PROGRAM MAIN_Simu
VAR
	bReset						AT %I*: BOOL;
(***** Cylinder states *****)
	bClampAtBase				AT %Q*: BOOL;					// True if clamp cylinder is in base position
	bClampAtWork				AT %Q*: BOOL;					// True if clamp cylinder is in work position
	bBarrierAtBase				AT %Q*: BOOL;					// True if barrier cylinder is in base position
	bBarrierAtWork				AT %Q*: BOOL;					// True if barrier cylinder is in work position
	bMetalAtBase				AT %Q*: BOOL;					// True if metal cylinder is in base position
	bMetalAtWork				AT %Q*: BOOL;					// True if metal cylinder is in work position
	bPlasticAtBase				AT %Q*: BOOL;					// True if plastic cylinder is in base position
	bPlasticAtWork				AT %Q*: BOOL;					// True if plastic cylinder is in work position
(***** Temperatures *****)
	lrClampTempCurrent			AT %Q*: LREAL;					// Current temperature of clamp cylinder
	lrClampTempMax				AT %Q*: LREAL;					// Maximum temperature of clamp cylinder
	lrClampTempMin				AT %Q*: LREAL;					// Minimum temperature of clamp cylinder
	lrBarrierTemp				AT %Q*: LREAL;					// Temperature of barrier cylinder

(***** Sensors to detect boxes *****)
	bBarrierSensor				AT %Q*: BOOL;					// True if barrier sensor detects a box
	bMetalSensor				AT %Q*: BOOL;					// True if metal sensor detects a metal box
	bPlasticSensor				AT %Q*: BOOL;					// True if plastic sensor detects a box

(* Position variables *)
	lrYClamp					AT %I*: LREAL;					// Y-Coordinate of clamp cylinder
	lrYBarrier					AT %I*: LREAL;					// Y-Coordinate of barrier cylinder
	lrYMetal					AT %I*: LREAL;					// Y-Coordinate of metal cylinder
	lrYPlastic					AT %I*: LREAL;					// Y-Coordinate of plastic cylinder
	lrBoxX						AT %I*: ARRAY[1..4] OF LREAL;	// X-Coordinates of boxes
	lrBoxY						AT %I*: ARRAY[1..4] OF LREAL;	// Y-Coordinates of boxes
	
	bTempUp						: BOOL;							// To raise temperature of clamp cylinder
	tonTemp						: TON;							// Timer to change temperature
END_VAR

// =========================================================
	// Resetting temperatures
	
IF bReset THEN
	lrClampTempCurrent := 0;
	lrBarrierTemp := 0;
END_IF

// =========================================================
	// Cylinder temperatures
	
A_Temperatures();

// =========================================================
	// Output variables
	
A_SetOutput();

// =========================================================

ACTION A_Temperatures:
// =========================================================
	// Temperature of cylinders
	
lrClampTempMax 		:= 60.5;
lrClampTempMin 		:= 9.4;
lrClampTempCurrent 	:= 10.7;

tonTemp( PT := T#1S );

IF NOT tonTemp.Q THEN
	tonTemp( IN := TRUE );
END_IF

IF lrBarrierTemp >= 55 THEN
	bTempUp := FALSE;
ELSIF lrBarrierTemp <=	10 THEN
	bTempUp := TRUE;
END_IF

IF tonTemp.Q THEN
	
	tonTemp( IN := FALSE );
	
	IF bTempUp THEN
		lrBarrierTemp := lrBarrierTemp + 1.2;
	ELSE
		lrBarrierTemp := lrBarrierTemp - 1.2;
	END_IF
END_IF

// =========================================================
END_ACTION

ACTION A_SetOutput:
// =========================================================
	// Cylinder feedback for base and work position
	
bClampAtWork 	:= (lrYClamp = 3.0);
bClampAtBase 	:= (lrYClamp = 0.0);
bBarrierAtWork 	:= (lrYBarrier = 63.0);
bBarrierAtBase 	:= (lrYBarrier = 0.0);
bMetalAtWork 	:= (lrYMetal < -72.9) AND (lrYMetal > -73.1);
bMetalAtBase 	:= (lrYMetal = 0.0);
bPlasticAtWork 	:= (lrYPlastic < -72.9) AND (lrYPlastic > -73.1);
bPlasticAtBase 	:= (lrYPlastic = 0.0);

// =========================================================
	// Sensor variables
	
bBarrierSensor := ( (lrBoxY[1] >= -5) AND (lrBoxX[1] > -1) AND (lrBoxX[1] < 60) )
				OR ( (lrBoxY[2] >= -5) AND (lrBoxX[2] > 59) AND (lrBoxX[2] < 120) )
				OR ( (lrBoxY[3] >= -5) AND (lrBoxX[3] > 119) AND (lrBoxX[3] < 180) )
				OR ( (lrBoxY[4] >= -5) AND (lrBoxX[4] > 179) AND (lrBoxX[4] < 240) );
				
bMetalSensor := ( (lrBoxY[1] >= -5) AND (lrBoxX[1] > 134) AND (lrBoxX[1] < 197) )
				OR ( (lrBoxY[4] >= -5) AND (lrBoxX[4] > 314) AND (lrBoxX[4] < 377) );
				
bPlasticSensor := ( (lrBoxY[1] >= -5) AND (lrBoxX[1] > 384) AND (lrBoxX[1] < 447) )
				OR ( (lrBoxY[2] >= -5) AND (lrBoxX[2] > 444) AND (lrBoxX[2] < 507) )
				OR ( (lrBoxY[3] >= -5) AND (lrBoxX[3] > 504) AND (lrBoxX[3] < 567) )
				OR ( (lrBoxY[4] >= -5) AND (lrBoxX[4] > 564) AND (lrBoxX[4] < 627) );

// =========================================================
END_ACTION

END_PROGRAM
